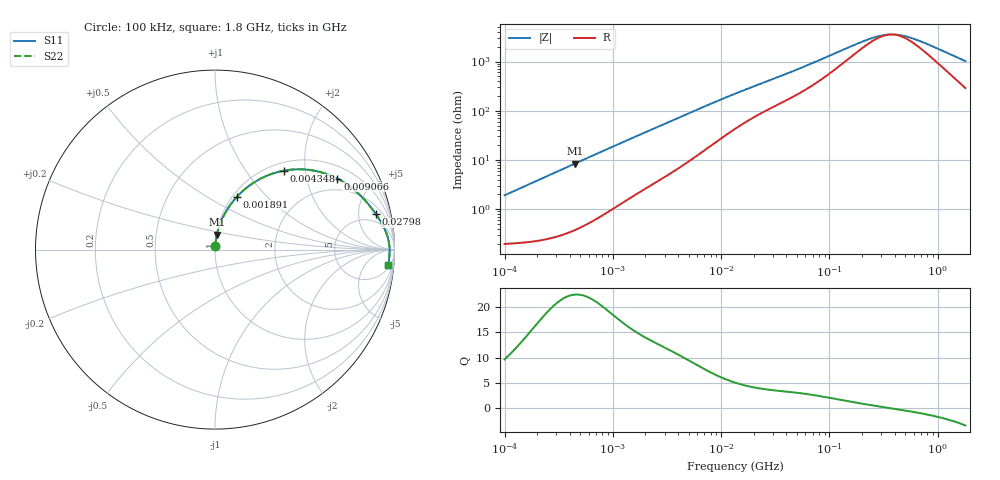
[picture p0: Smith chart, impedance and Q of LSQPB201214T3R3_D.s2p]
! LSQPB201214T3R3_D  S-PARAMETER MODEL  ( General Type )
! Model Generated by TAIYO YUDEN Corporation (http://www.ty-top.com)
! Version 1.0
! TAIYO YUDEN Control No. 100901NG22SB-FKC
! Copyright(c) 2010 TAIYO YUDEN CO.,LTD. All Rights Reserved.
! Product Description (link to TY-COMPAS)
! https://ds.yuden.co.jp/TYCOMPAS/or/detail?pn=LSQPB201214T3R3MD&u=M
! Products Name : Inductors
! Characteristics :
!  Inductance : 3.3 uH , SRF(min) : 300 MHz , DC Resistance(max) : 0.221 Ohm
!  Rated Current : Saturation :800 mA , Temp Rise : 870 mA (40 degC)
!  Case Size : 2.0 x 1.25 / 0.079 x 0.049 [mm/inch] , Thickness : 1.4 / 0.056 [mm/inch]
!  (Conditions: Temperature = 25 degC , DC Bias Current/Voltage = 0A / 0V)
! External Node Assignments :
!  1  o---GGG---o  2
! GND o---------o GND
! Frequency Range : 0.1MHz  -  1800MHz  [ 402 STEP ]
# MHz S RI R 50
! Freq[MHz].  S11 Real  S11 Imag  S21 Real  S21 Imag  S12 Real  S12 Imag  S22 Real  S22 Imag
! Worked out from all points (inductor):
!   401 points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, 100 kHz to 1.8 GHz, reference 50 ohm
!   read as one part in series: L = 3.02 uH near 105 kHz
!   highest Q = 22.5 at 445.6 kHz (marker M1), where L = 3.01 uH
!   self-resonance near 372.1 MHz
!   S11 on the Smith chart (normalised r, x): 100 kHz: 1.00, +0.04; 1.891 MHz: 1.05, +0.69; 4.348 MHz: 1.15, +1.54; 9.066 MHz: 1.47, +3.07; 27.98 MHz: 3.19, +7.99; 1.8 GHz: 7, -20
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0.1  0.00232 0.0189  0.9977 -0.0189  0.9977 -0.0189  0.00232 0.0189
0.229984  0.00426 0.0433  0.9957 -0.0433  0.9957 -0.0433  0.00426 0.0433
0.445583  0.0107 0.0829  0.9893 -0.0829  0.9893 -0.0829  0.0107 0.0829
0.516129  0.0136 0.0956  0.9864 -0.0956  0.9864 -0.0956  0.0136 0.0956
1.076226  0.0484 0.1886  0.9516 -0.1886  0.9516 -0.1886  0.0484 0.1886
1.890522  0.1233 0.2956  0.8767 -0.2956  0.8767 -0.2956  0.1233 0.2956
2.66389  0.2064 0.367  0.7936 -0.367  0.7936 -0.367  0.2064 0.367
3.320932  0.2786 0.4071  0.7214 -0.4071  0.7214 -0.4071  0.2786 0.4071
4.347904  0.3845 0.4399  0.6155 -0.4399  0.6155 -0.4399  0.3845 0.4399
6.126528  0.5315 0.4431  0.4685 -0.4431  0.4685 -0.4431  0.5315 0.4431
9.066201  0.6817 0.3955  0.3183 -0.3955  0.3183 -0.3955  0.6817 0.3955
13.41641  0.7888 0.3215  0.2112 -0.3215  0.2112 -0.3215  0.7888 0.3215
18.90474  0.8503 0.2579  0.1497 -0.2579  0.1497 -0.2579  0.8503 0.2579
27.97575  0.8972 0.1964  0.1028 -0.1964  0.1028 -0.1964  0.8972 0.1964
69.24595  0.9542 0.0932  0.0458 -0.0932  0.0458 -0.0932  0.9542 0.0932
218.9722  0.9714 0.0212  0.0286 -0.0212  0.0286 -0.0212  0.9714 0.0212
286.6876  0.9722 0.0101  0.0278 -0.0101  0.0278 -0.0101  0.9722 0.0101
357.3983  0.9725 0.00154  0.0275 -0.00154  0.0275 -0.00154  0.9725 0.00154
456.5984  0.9726 -0.00793  0.0274 0.00793  0.0274 0.00793  0.9726 -0.00793
597.7978  0.9725 -0.0189  0.0275 0.0189  0.0275 0.0189  0.9725 -0.0189
821.96  0.9717 -0.0338  0.0283 0.0338  0.0283 0.0338  0.9717 -0.0338
1800  0.9648 -0.0884  0.0352 0.0884  0.0352 0.0884  0.9648 -0.0884
